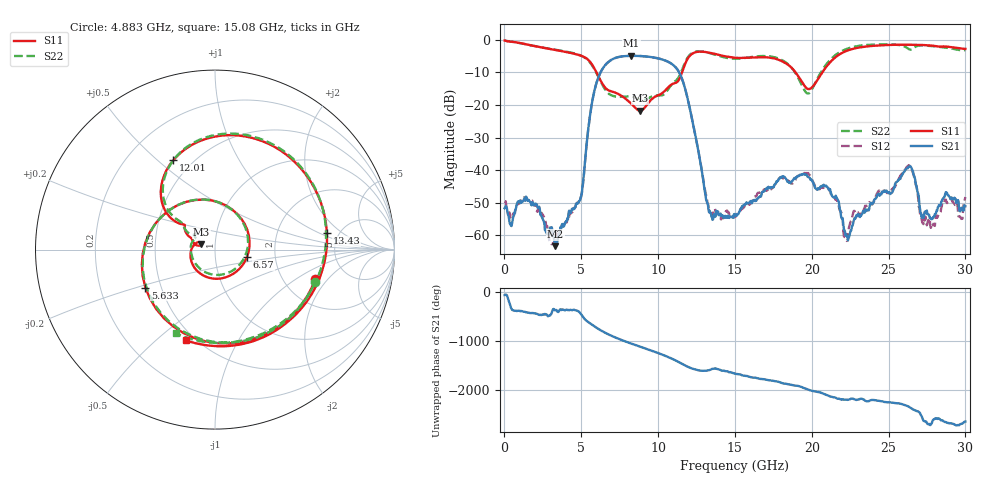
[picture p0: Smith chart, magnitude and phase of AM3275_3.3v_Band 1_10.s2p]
!Keysight Technologies,N5245B,MY58422270,A.16.20.02
!Date: Thursday, March 27, 2025 01:45:54
!Correction: S11(C  2-Port  )
!S21(C  2-Port  )
!S12(C  2-Port  )
!S22(C  2-Port  )
!S2P File: Measurements: S11, S21, S12, S22:
# Hz S  dB  R 50
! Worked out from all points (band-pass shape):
!   801 points, 10 MHz to 30 GHz, reference 50 ohm
!   highest |S21| = -4.87 dB at 8.257 GHz (marker M1); lowest = -63.4 dB at 3.309 GHz (marker M2)
!   |S21| within 3 dB of the highest: 6.535 GHz to 11.02 GHz (4.488 GHz wide, 51.1 % of centre)
!   lowest |S11| = -21.7 dB at 8.82 GHz (marker M3), VSWR 1.18, Z = 42.8 + j2.54 ohm
!   |S11| at or under -10 dB: 5.99 GHz to 11.56 GHz (5.566 GHz wide, 63.4 % of centre); 18.95 GHz to 20.68 GHz (1.731 GHz wide, 8.74 % of centre)
!   |S22| runs from -18.5 to -0.2 dB; largest |S21 - S12| = 0.0056
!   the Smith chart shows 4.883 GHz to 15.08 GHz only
!   S11 on the Smith chart (normalised r, x): 4.883 GHz: 2.97, -1.49; 5.633 GHz: 0.41, -0.21; 6.57 GHz: 1.43, -0.12; 12.01 GHz: 0.40, +0.56; 13.43 GHz: 4.00, +1.23; 15.08 GHz: 0.45, -0.63
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1e7  -0.16 -4.9  -51.73 -54.6  -49.57 85.2  -0.21 -5.6
1.172112e9  -1.10 -96.5  -49.76 -25.9  -48.67 -25.9  -1.13 -97.0
3.3089e9  -3.08 122.1  -63.38 -0.9  -59.92 -44.3  -3.00 120.9
4.883375e9  -4.69 -16.6  -49.57 -44.1  -49.37 -47.9  -4.64 -18.2
5.033325e9  -4.93 -37.8  -47.14 -104.5  -47.19 -107.3  -4.94 -39.8
5.633125e9  -7.10 -151.4  -21.14 74.3  -21.19 73.9  -7.34 -156.5
6.570312e9  -14.75 -12.8  -7.67 -107.5  -7.67 -107.5  -15.36 -13.2
7.2076e9  -16.18 -127.5  -5.55 159.4  -5.55 159.3  -17.38 -123.9
8.25725e9  -19.63 156.8  -4.87 33.0  -4.87 32.9  -17.37 165.0
8.819562e9  -21.74 158.9  -4.93 -28.8  -4.93 -28.8  -18.29 149.6
1.001916e10  -16.94 155.3  -5.68 -162.7  -5.68 -162.8  -17.11 140.7
1.08064e10  -13.92 146.3  -7.12 97.3  -7.11 97.3  -14.17 146.5
1.2006e10  -5.19 114.9  -19.77 -91.8  -19.79 -91.7  -4.88 110.8
1.343052e10  -4.02 8.5  -53.15 -140.3  -53.23 -134.7  -4.14 5.0
1.5005e10  -5.47 -102.3  -53.72 136.7  -54.14 139.8  -5.76 -109.5
1.507998e10  -5.50 -107.6  -53.66 132.9  -54.20 129.0  -5.76 -114.9
1.755415e10  -5.68 106.2  -44.77 -13.2  -44.66 -16.8  -5.30 102.5
2.002832e10  -14.52 -106.9  -43.22 144.1  -43.05 142.5  -15.06 -121.1
2.22026e10  -3.47 119.7  -60.03 -37.6  -60.88 8.3  -2.88 114.9
2.501416e10  -1.55 39.2  -46.84 -88.6  -47.15 -88.4  -1.33 36.2
2.748834e10  -1.64 -22.4  -52.41 -151.6  -56.96 147.4  -1.76 -22.2
3e10  -2.75 -107.9  -51.08 -122.2  -48.28 -152.1  -3.13 -110.5
